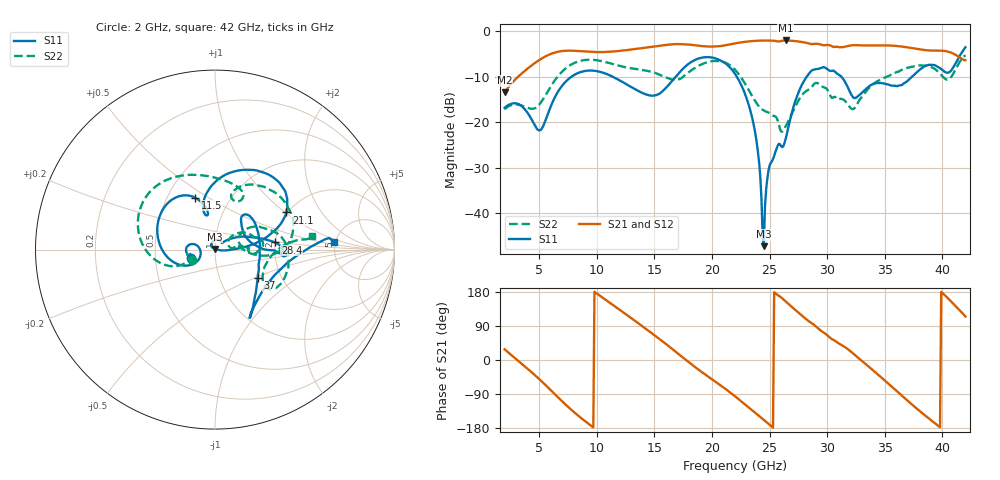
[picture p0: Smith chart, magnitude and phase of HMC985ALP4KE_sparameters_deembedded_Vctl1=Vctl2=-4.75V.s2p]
!s2p File: Measurements: S11, S21, S12, S22
# GHz S dB R 50.0
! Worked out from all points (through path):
!   401 points, 2 GHz to 42 GHz, reference 50 ohm
!   highest |S21| = -2.06 dB at 26.4 GHz (marker M1); lowest = -13.4 dB at 2 GHz (marker M2)
!   lowest |S11| = -47.2 dB at 24.5 GHz (marker M3), VSWR 1.01, Z = 49.8 + j0.401 ohm
!   |S11| at or under -10 dB: start of sweep to 7.814 GHz; 22.15 GHz to 28.23 GHz (6.081 GHz wide, 24.1 % of centre); 31.22 GHz to 37.38 GHz (6.159 GHz wide, 18 % of centre)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
!   |S22| runs from -22.1 to -5.3 dB; largest |S21 - S12| = 0.00095
!   S11 on the Smith chart (normalised r, x): 2 GHz: 0.76, -0.07; 11.5 GHz: 0.69, +0.44; 21.1 GHz: 1.97, +1.02; 28.4 GHz: 2.00, +0.18; 37 GHz: 1.51, -0.52; 42 GHz: 4.83, +0.76
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2  -16.86 -161.8  -13.43 28.2  -13.44 28.2  -17.16 -155.6
5  -21.81 -172.8  -6.38 -50.2  -6.38 -50.2  -16.16 -159.9
6.3  -14.86 -150.4  -4.76 -88.4  -4.76 -88.4  -11.02 -161.7
8.7  -8.92 150.3  -4.44 -154.6  -4.44 -154.6  -6.46 151.2
11.5  -10.18 111.0  -4.47 143.1  -4.47 143.1  -7.31 105.0
13.6  -13.13 101.2  -3.85 97.1  -3.85 97.1  -8.41 75.6
15.4  -13.80 106.0  -3.25 56.3  -3.25 56.4  -9.52 62.0
17.9  -7.32 80.2  -2.94 -3.7  -2.94 -3.7  -9.19 72.0
21.1  -6.97 27.5  -3.15 -74.5  -3.15 -74.5  -6.87 15.9
22  -9.37 17.0  -2.71 -95.7  -2.71 -95.7  -8.47 0.5
23.6  -20.29 0.2  -2.18 -135.4  -2.18 -135.4  -14.76 -4.4
24.5  -47.22 112.5  -2.08 -158.1  -2.08 -158.1  -17.42 8.2
25  -29.54 131.5  -2.10 -170.8  -2.10 -170.8  -18.00 11.1
26.4  -23.63 41.6  -2.06 154.5  -2.06 154.5  -20.89 32.9
28.4  -9.41 6.7  -2.71 102.5  -2.71 102.5  -12.86 18.1
28.7  -8.59 1.8  -2.85 96.2  -2.86 96.2  -12.17 16.2
30.7  -8.97 -3.2  -3.45 50.4  -3.45 50.4  -14.46 2.0
32.5  -14.61 31.9  -3.10 10.6  -3.09 10.6  -16.45 27.7
35.4  -11.81 19.1  -3.17 -64.9  -3.16 -64.9  -9.78 19.3
37  -10.88 -33.9  -3.58 -108.1  -3.58 -108.0  -8.06 4.8
39.8  -8.14 -57.4  -4.29 -177.6  -4.29 -177.6  -9.32 -35.8
42  -3.55 3.8  -6.37 114.6  -6.38 114.7  -5.30 8.2
